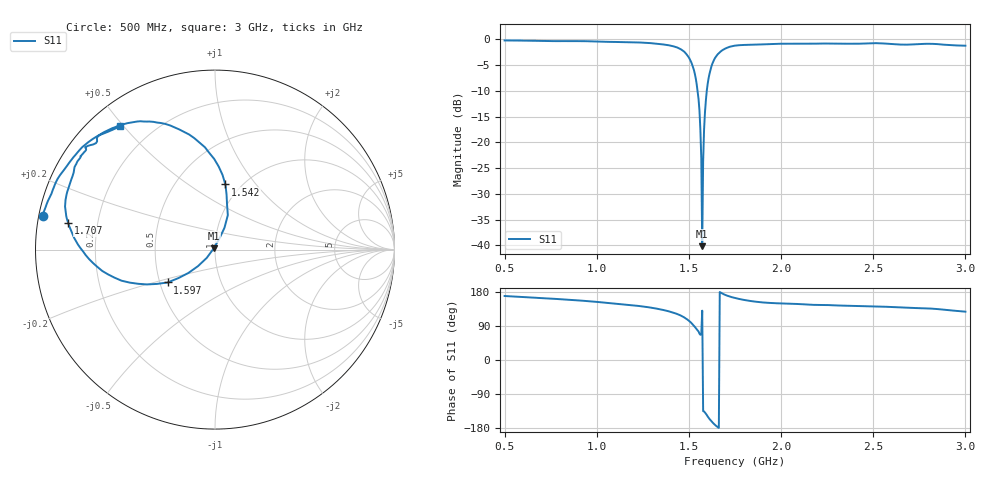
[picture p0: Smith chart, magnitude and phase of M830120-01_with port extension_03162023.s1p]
# Hz S RI R 50
! CMT, M5090, 19127454, 21.2.4/2
! Date: 3/16/2023 5:30:10 PM
! Data: Format (Calibration Info)
! Freq	S11:Re/Im(F2 Pxt)
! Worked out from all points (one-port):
!   500 points, 500 MHz to 3 GHz, reference 50 ohm
!   lowest |S11| = -40.2 dB at 1.572 GHz (marker M1), VSWR 1.02, Z = 49.4 + j0.741 ohm
!   |S11| at or under -10 dB: 1.547 GHz to 1.597 GHz (49.98 MHz wide, 3.18 % of centre)
!   S11 on the Smith chart (normalised r, x): 500 MHz: 0.01, +0.10; 1.542 GHz: 0.85, +0.71; 1.597 GHz: 0.55, -0.22; 1.707 GHz: 0.09, +0.09; 3 GHz: 0.09, +0.49
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5e8  -0.9589 0.1887
8.156313e8  -0.9051 0.3297
1.126253e9  -0.7975 0.5032
1.321643e9  -0.6529 0.6342
1.441884e9  -0.4152 0.7151
1.502004e9  -0.1438 0.6411
1.527054e9  -0.00429 0.505
1.542084e9  0.0578 0.363
1.552104e9  0.0668 0.2563
1.557114e9  0.0714 0.1919
1.562124e9  0.0529 0.1218
1.567134e9  0.0257 0.0639
1.572144e9  -0.00634 0.00751
1.577154e9  -0.046 -0.0462
1.582164e9  -0.0949 -0.0923
1.587174e9  -0.1482 -0.1302
1.597194e9  -0.2639 -0.183
1.617234e9  -0.4746 -0.184
1.642285e9  -0.6566 -0.0953
1.672345e9  -0.7635 0.028
1.707415e9  -0.8172 0.1472
1.752505e9  -0.8348 0.2504
1.882766e9  -0.7939 0.4087
2.063126e9  -0.7716 0.4798
2.378758e9  -0.7239 0.5477
2.689379e9  -0.6578 0.6002
2.819639e9  -0.6464 0.6352
3e9  -0.5292 0.6894
